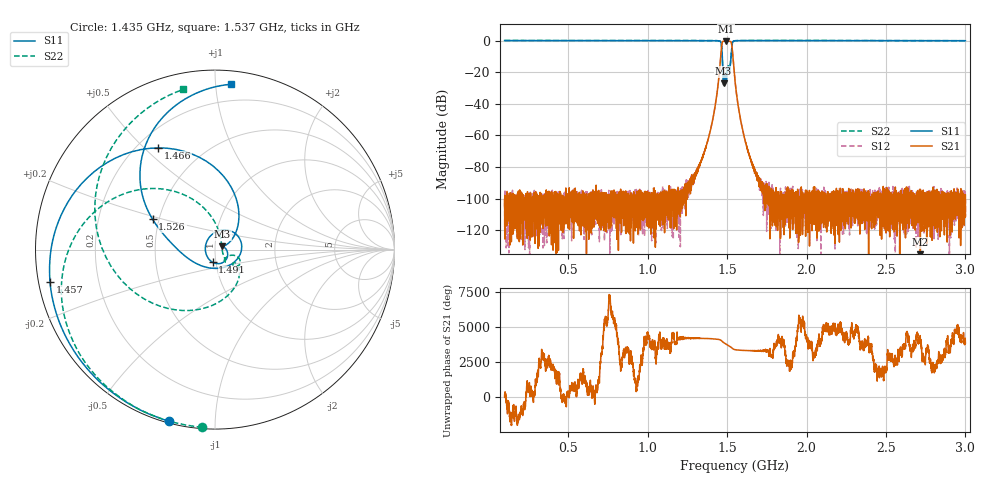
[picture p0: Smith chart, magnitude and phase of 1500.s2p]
# Hz S DB R 50
! Planar, S50180, 20087770, 20.1.2/1
! Date: 23.06.2021 14:43:37
! Data: Format (Calibration Info)
! Freq	S11:dB/Ang(F2)	S21:dB/Ang(F2)	S12:dB/Ang(F2)	S22:dB/Ang(F2)
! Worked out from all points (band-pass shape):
!   8991 points, 100 MHz to 3 GHz, reference 50 ohm
!   highest |S21| = -0.37 dB at 1.494 GHz (marker M1); lowest = -139.6 dB at 2.716 GHz (marker M2)
!   |S21| within 3 dB of the highest: 1.466 GHz to 1.531 GHz (64.52 MHz wide, 4.31 % of centre)
!   lowest |S11| = -27.1 dB at 1.478 GHz (marker M3), VSWR 1.09, Z = 54.2 + j1.93 ohm
!   |S11| at or under -10 dB: 1.47 GHz to 1.525 GHz (55.13 MHz wide, 3.68 % of centre)
!   |S22| runs from -28.1 to 0.0 dB; largest |S21 - S12| = 0.0027
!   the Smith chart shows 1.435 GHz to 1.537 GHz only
!   S11 on the Smith chart (normalised r, x): 1.435 GHz: 0.01, -0.77; 1.457 GHz: 0.03, -0.10; 1.466 GHz: 0.28, +0.55; 1.491 GHz: 0.97, -0.14; 1.526 GHz: 0.46, +0.18; 1.537 GHz: 0.09, +1.10
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1e8  0.02 154.0  -104.39 -3.2  -102.58 27.5  0.01 150.2
3.122581e8  -0.03 104.1  -98.19 139.1  -102.48 142.4  0.00 95.4
5.835484e8  -0.01 55.0  -101.22 -76.7  -101.25 -75.7  0.01 45.7
1.066774e9  0.00 -7.9  -104.12 147.6  -98.80 -38.2  0.04 -13.4
1.321613e9  -0.01 -45.4  -78.89 -138.6  -79.05 -140.5  0.00 -46.9
1.386452e9  -0.03 -65.9  -60.31 -155.4  -60.31 -156.1  0.02 -63.4
1.434839e9  -0.09 -105.1  -34.88 168.4  -34.89 168.4  -0.06 -94.1
1.457419e9  -0.57 -169.0  -13.52 110.1  -13.53 110.0  -0.46 -144.4
1.465806e9  -3.74 119.3  -3.58 43.9  -3.58 43.8  -3.60 156.8
1.477742e9  -27.11 23.7  -0.43 -75.0  -0.44 -75.1  -27.95 -3.4
1.49129e9  -22.88 -100.3  -0.38 -170.5  -0.39 -170.6  -21.43 -53.5
1.493871e9  -24.90 -144.3  -0.37 172.6  -0.38 172.5  -22.33 -45.2
1.506774e9  -16.47 24.2  -0.46 88.7  -0.46 88.7  -15.97 -28.7
1.526452e9  -8.27 154.1  -1.31 -66.3  -1.32 -66.4  -8.68 -112.8
1.537419e9  -0.67 84.4  -11.09 -173.9  -11.09 -174.0  -0.82 101.2
1.55e9  -0.14 44.3  -25.38 136.2  -25.38 136.2  -0.14 43.4
1.598387e9  -0.02 -2.5  -56.78 85.2  -56.87 85.0  -0.02 -9.8
1.668065e9  -0.02 -24.9  -80.37 61.5  -80.15 59.4  0.02 -31.1
2.033548e9  -0.04 -68.2  -109.25 -121.7  -104.29 -173.0  -0.01 -70.5
2.516774e9  -0.07 -105.8  -103.57 121.9  -100.44 -107.2  -0.05 -104.9
2.716452e9  -0.08 -120.1  -139.63 -87.0  -101.47 -136.7  -0.06 -118.2
3e9  -0.10 -141.2  -97.73 -116.4  -99.86 -36.6  -0.09 -137.9
